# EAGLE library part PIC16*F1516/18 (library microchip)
28/40/44-Pin Flash Microcontrollers with nanoWatt XLP Technology PIC16F1516/1518 AND PIC16LF1516/1518 Source: www.microchip.com PIC16F1516.pdf
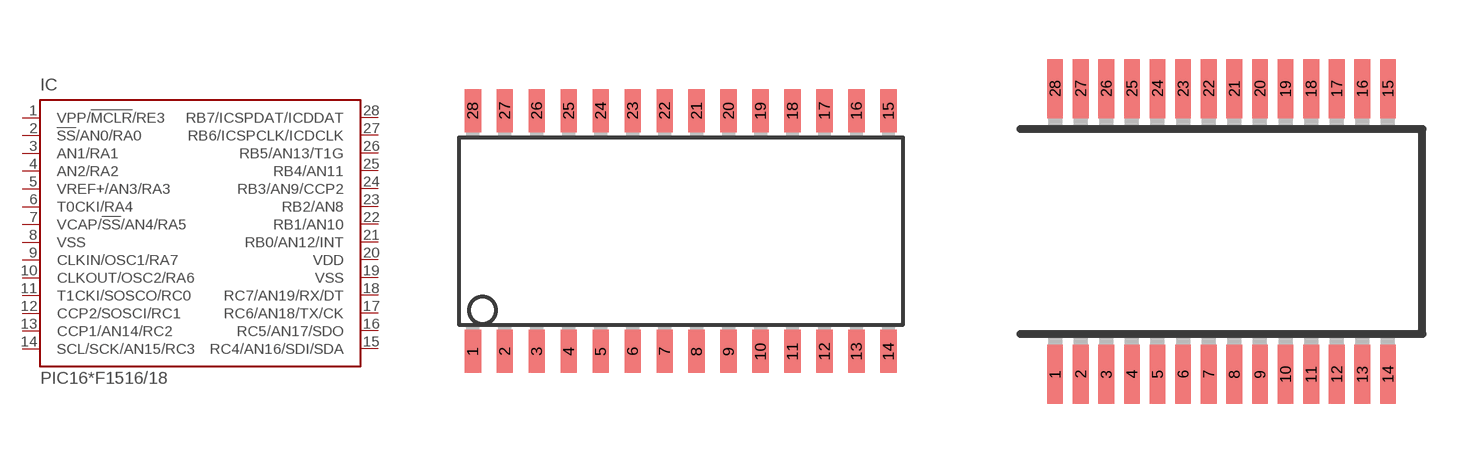
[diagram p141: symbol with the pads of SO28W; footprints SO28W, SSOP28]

Designator prefix IC

## PIC16F1516/18SO, PIC16LF1516/18SO  [SO28W]
1  VPP/!MCLR!/RE3
2  !SS!/AN0/RA0
3  AN1/RA1
4  AN2/RA2
5  VREF+/AN3/RA3
6  T0CKI/RA4
7  VCAP/!SS!/AN4/RA5
8  VSS  pwr
9  CLKIN/OSC1/RA7
10  CLKOUT/OSC2/RA6
11  T1CKI/SOSCO/RC0
12  CCP2/SOSCI/RC1
13  CCP1/AN14/RC2
14  SCL/SCK/AN15/RC3
15  RC4/AN16/SDI/SDA
16  RC5/AN17/SDO
17  RC6/AN18/TX/CK
18  RC7/AN19/RX/DT
19  VSS  pwr
20  VDD  pwr
21  RB0/AN12/INT
22  RB1/AN10
23  RB2/AN8
24  RB3/AN9/CCP2
25  RB4/AN11
26  RB5/AN13/T1G
27  RB6/ICSPCLK/ICDCLK
28  RB7/ICSPDAT/ICDDAT

## PIC16F1516/18SS, PIC16LF1516/18SS  [SSOP28]
Pads as for SO28W

## PIC16F1516/18P, PIC16LF1516/18P  [DIL28-3]
Pads as for SO28W

## PIC16F1516/18ML  [UQFN28_4X4MM]
1  AN2/RA2
2  VREF+/AN3/RA3
3  T0CKI/RA4
4  VCAP/!SS!/AN4/RA5
5  VSS  pwr
6  CLKIN/OSC1/RA7
7  CLKOUT/OSC2/RA6
8  T1CKI/SOSCO/RC0
9  CCP2/SOSCI/RC1
10  CCP1/AN14/RC2
11  SCL/SCK/AN15/RC3
12  RC4/AN16/SDI/SDA
13  RC5/AN17/SDO
14  RC6/AN18/TX/CK
15  RC7/AN19/RX/DT
16  VSS  pwr
17  VDD  pwr
18  RB0/AN12/INT
19  RB1/AN10
20  RB2/AN8
21  RB3/AN9/CCP2
22  RB4/AN11
23  RB5/AN13/T1G
24  RB6/ICSPCLK/ICDCLK
25  RB7/ICSPDAT/ICDDAT
26  VPP/!MCLR!/RE3
27  !SS!/AN0/RA0
28  AN1/RA1

## Footprint SO28W (pad centres in mm)
28-Lead Plastic Small Outline (SO) Wide, 300 mil Body (SOIC) Source: http://ww1.microchip.com/downloads/en/devicedoc/39632c.pdf
smd 0.65 x 1.7: 1 -7.62,-4.78; 2 -6.35,-4.78; 3 -5.08,-4.78; 4 -3.81,-4.78; 5 -2.54,-4.78; 6 -1.27,-4.78; 7 0,-4.78; 8 1.27,-4.78; 9 2.54,-4.78; 10 3.81,-4.78; 11 5.08,-4.78; 12 6.35,-4.78; 13 7.62,-4.78; 14 8.89,-4.78; 15 8.89,4.78; 16 7.62,4.78; 17 6.35,4.78; 18 5.08,4.78; 19 3.81,4.78; 20 2.54,4.78; 21 1.27,4.78; 22 0,4.78; 23 -1.27,4.78; 24 -2.54,4.78; 25 -3.81,4.78; 26 -5.08,4.78; 27 -6.35,4.78; 28 -7.62,4.78

## Footprint SSOP28 (pad centres in mm)
Shrink Small Outline Package package type SS
smd 0.4 x 1.5: 1 -4.225,-3.625; 2 -3.575,-3.625; 3 -2.925,-3.625; 4 -2.275,-3.625; 5 -1.625,-3.625; 6 -0.975,-3.625; 7 -0.325,-3.625; 8 0.325,-3.625; 9 0.975,-3.625; 10 1.625,-3.625; 11 2.275,-3.625; 12 2.925,-3.625; 13 3.575,-3.625; 14 4.225,-3.625; 15 4.225,3.625; 16 3.575,3.625; 17 2.925,3.625; 18 2.275,3.625; 19 1.625,3.625; 20 0.975,3.625; 21 0.325,3.625; 22 -0.325,3.625; 23 -0.975,3.625; 24 -1.625,3.625; 25 -2.275,3.625; 26 -2.925,3.625; 27 -3.575,3.625; 28 -4.225,3.625

## Footprint DIL28-3 (pad centres in mm)
Dual In Line package type P
drill 0.813 long: 1 -16.51,-3.81; 2 -13.97,-3.81; 3 -11.43,-3.81; 4 -8.89,-3.81; 5 -6.35,-3.81; 6 -3.81,-3.81; 7 -1.27,-3.81; 8 1.27,-3.81; 9 3.81,-3.81; 10 6.35,-3.81; 11 8.89,-3.81; 12 11.43,-3.81; 13 13.97,-3.81; 14 16.51,-3.81; 15 16.51,3.81; 16 13.97,3.81; 17 11.43,3.81; 18 8.89,3.81; 19 6.35,3.81; 20 3.81,3.81; 21 1.27,3.81; 22 -1.27,3.81; 23 -3.81,3.81; 24 -6.35,3.81; 25 -8.89,3.81; 26 -11.43,3.81; 27 -13.97,3.81; 28 -16.51,3.81

## Footprint UQFN28_4X4MM (pad centres in mm)
28-Lead Platic Ultra Thin Quad Flat, No Lead Package (MV) - 4x4x0.5 mm Body [UQFN] Source: PIC16F1516.pdf
smd 0.65 x 0.25: 1 -1.8,1.2; 2 -1.8,0.8; 3 -1.8,0.4; 4 -1.8,0; 5 -1.8,-0.4; 6 -1.8,-0.8; 7 -1.8,-1.2; 15 1.8,-1.2; 16 1.8,-0.8; 17 1.8,-0.4; 18 1.8,0; 19 1.8,0.4; 20 1.8,0.8; 21 1.8,1.2
smd 0.25 x 0.65: 8 -1.2,-1.8; 9 -0.8,-1.8; 10 -0.4,-1.8; 11 0,-1.8; 12 0.4,-1.8; 13 0.8,-1.8; 14 1.2,-1.8; 22 1.2,1.8; 23 0.8,1.8; 24 0.4,1.8; 25 0,1.8; 26 -0.4,1.8; 27 -0.8,1.8; 28 -1.2,1.8
smd 2.75 x 2.75: TH 0,0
